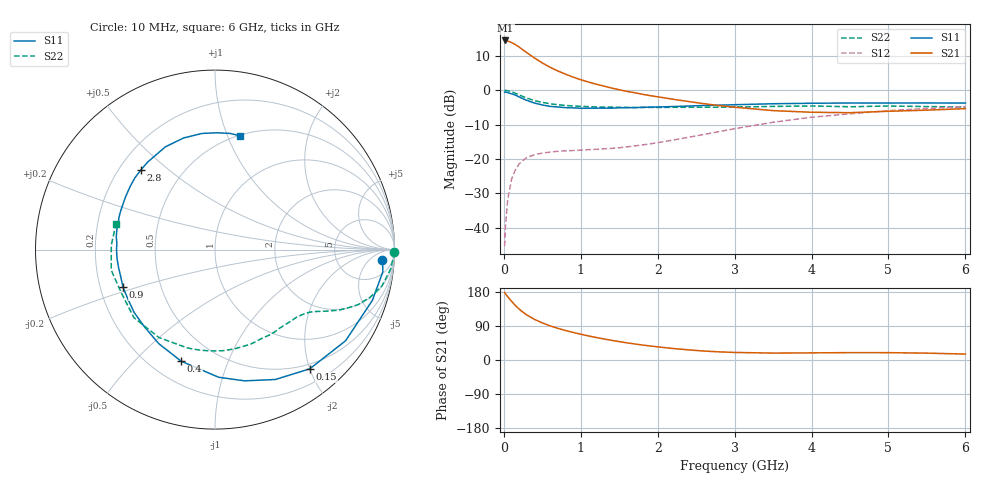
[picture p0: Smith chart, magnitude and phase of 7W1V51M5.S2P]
! Infineon Technologies  Discrete & RF Semiconductors
! BFS17W
! Si NPN RF Bipolar Junction Transistor in SOT323
! VCE = 1.5 V  IC = 1.5 mA
! Common Emitter S-Parameters:  August  1999
# GHz  S  MA  R  50
!  f  S11  S21  S12  S22
! GHz  MAG  ANG  MAG  ANG  MAG  ANG  MAG  ANG
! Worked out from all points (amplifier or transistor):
!   36 points, 10 MHz to 6 GHz, reference 50 ohm
!   highest |S21| = 14.5 dB at 20 MHz (marker M1)
!   |S21| within 3 dB of that: start of sweep to 264.1 MHz
!   unconditionally stable (mu >= 1): 872.4 MHz to end of sweep
!   at 250 MHz: K = 0.33, MSG = 16.0 dB, |S12| = -20.4 dB
!   at 1.4 GHz: K = 1.36, MAG = 5.2 dB, |S12| = -16.9 dB
!   at 6 GHz: K = 1.12, MAG = -2.4 dB, |S12| = -4.8 dB
!   S11 on the Smith chart (normalised r, x): 10 MHz: 16, -15; 150 MHz: 0.42, -2.00; 400 MHz: 0.32, -0.69; 900 MHz: 0.30, -0.18; 2.8 GHz: 0.29, +0.41; 6 GHz: 0.50, +1.11
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0.01  0.9349 -3.5  5.257 178.2  0.0054 83.5  0.9986 -0.8
0.02  0.9435 -7.5  5.289 174.9  0.0101 88.1  0.9946 -2.6
0.05  0.9212 -17.9  5.186 167.0  0.0257 80.3  0.9837 -6.5
0.1  0.8874 -34.9  4.938 155.1  0.0505 70.7  0.9513 -12.4
0.15  0.8486 -51.5  4.604 143.7  0.0696 61.7  0.9026 -17.2
0.2  0.798 -65.1  4.24 134.2  0.085 55.4  0.8544 -21.0
0.25  0.7496 -77.3  3.843 126.0  0.0956 49.1  0.8068 -23.8
0.3  0.7114 -88.4  3.505 118.8  0.105 45.3  0.7691 -26.0
0.4  0.6495 -106.9  2.931 107.0  0.1158 39.1  0.7055 -29.1
0.5  0.6103 -121.0  2.492 97.9  0.1217 35.3  0.6651 -31.2
0.6  0.582 -132.9  2.158 90.2  0.1259 33.1  0.6353 -33.2
0.7  0.5703 -142.3  1.91 83.7  0.1294 32.6  0.6155 -35.3
0.9  0.5539 -157.7  1.551 72.8  0.1326 32.2  0.5894 -39.9
1.1  0.5466 -169.8  1.314 63.4  0.1366 33.9  0.5767 -45.0
1.6  0.5583 168.3  0.961 45.3  0.1499 41.7  0.5613 -59.7
2.2  0.5788 149.3  0.739 30.3  0.1886 51.9  0.5638 -79.0
2.8  0.6062 132.8  0.597 21.5  0.2502 55.7  0.5665 -99.3
3.5  0.6358 115.8  0.505 18.3  0.3418 52.9  0.581 -122.5
4  0.6461 105.7  0.478 18.8  0.4047 47.5  0.5898 -140.1
4.5  0.6512 96.3  0.471 19.5  0.4531 41.4  0.5748 -155.7
5.5  0.6526 82.8  0.513 18.1  0.5418 29.8  0.5782 177.5
6  0.6499 77.7  0.54 15.6  0.5768 24.2  0.57 165.6
